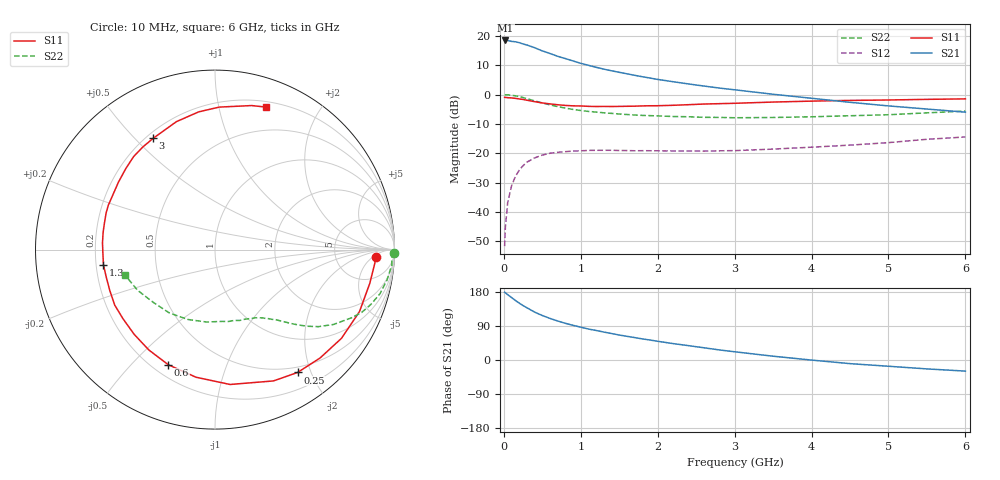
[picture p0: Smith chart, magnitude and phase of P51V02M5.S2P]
! SIEMENS Small Signal Semiconductors
! BFP183
! Si NPN RF Bipolar Junction Transistor in SOT143
! VCE = 1 V  IC = 2.5 mA
! Common Emitter S-Parameters:  March  1996
# GHz  S  MA  R  50
!  f  S11  S21  S12  S22
! GHz  MAG  ANG  MAG  ANG  MAG  ANG  MAG  ANG
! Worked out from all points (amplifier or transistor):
!   36 points, 10 MHz to 6 GHz, reference 50 ohm
!   highest |S21| = 18.4 dB at 20 MHz (marker M1)
!   |S21| within 3 dB of that: start of sweep to 448.6 MHz
!   unconditionally stable (mu >= 1): 1.912 GHz to end of sweep
!   at 250 MHz: K = 0.14, MSG = 20.7 dB, |S12| = -24.3 dB
!   at 1.4 GHz: K = 0.76, MSG = 13.6 dB, |S12| = -19.0 dB
!   at 6 GHz: K = 1.07, MAG = 2.6 dB, |S12| = -14.5 dB
!   S11 on the Smith chart (normalised r, x): 10 MHz: 16, -6; 250 MHz: 0.42, -1.80; 600 MHz: 0.26, -0.64; 1.3 GHz: 0.23, -0.07; 3 GHz: 0.23, +0.57; 6 GHz: 0.25, +1.39
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0.01  0.8958 -2.5  8.258 178.8  0.0026 86.7  0.9964 -1.0
0.02  0.8936 -4.9  8.357 177.5  0.0055 88.8  0.9872 -2.0
0.05  0.8829 -12.2  8.353 172.3  0.0144 85.6  0.9888 -5.1
0.15  0.8609 -35.0  7.935 157.1  0.0401 70.2  0.9513 -15.0
0.2  0.8411 -45.9  7.669 150.1  0.0513 65.0  0.9213 -19.3
0.25  0.8248 -56.1  7.273 143.6  0.0612 59.3  0.8889 -23.2
0.3  0.8009 -66.0  6.993 137.8  0.0704 54.6  0.8508 -26.5
0.4  0.7562 -83.6  6.287 126.4  0.0831 46.4  0.7808 -32.3
0.5  0.7189 -98.5  5.548 117.4  0.0929 39.3  0.7184 -36.7
0.6  0.6921 -112.1  5.008 109.7  0.0998 34.0  0.6669 -39.8
0.7  0.6698 -123.4  4.487 102.9  0.1036 29.8  0.6229 -42.3
0.8  0.6525 -133.6  4.101 96.8  0.1063 26.2  0.5871 -44.4
0.9  0.6413 -143.0  3.735 91.5  0.1086 23.5  0.557 -46.2
1.1  0.6291 -158.7  3.15 81.7  0.1116 18.7  0.5158 -49.1
1.3  0.6273 -172.1  2.71 73.7  0.1122 15.2  0.4878 -52.1
1.6  0.6306 171.4  2.258 62.5  0.111 12.5  0.4569 -56.3
2.2  0.6558 145.3  1.655 43.3  0.109 11.3  0.4221 -66.7
3  0.7092 119.1  1.205 21.7  0.1106 14.1  0.402 -84.3
3.5  0.7445 106.8  1.011 10.0  0.1175 16.6  0.4062 -96.7
4.5  0.7943 88.3  0.737 -9.6  0.1373 18.6  0.435 -125.8
5.5  0.8278 75.8  0.566 -23.5  0.1726 17.3  0.4874 -152.3
6  0.8437 70.2  0.501 -29.3  0.189 14.0  0.5218 -164.3
